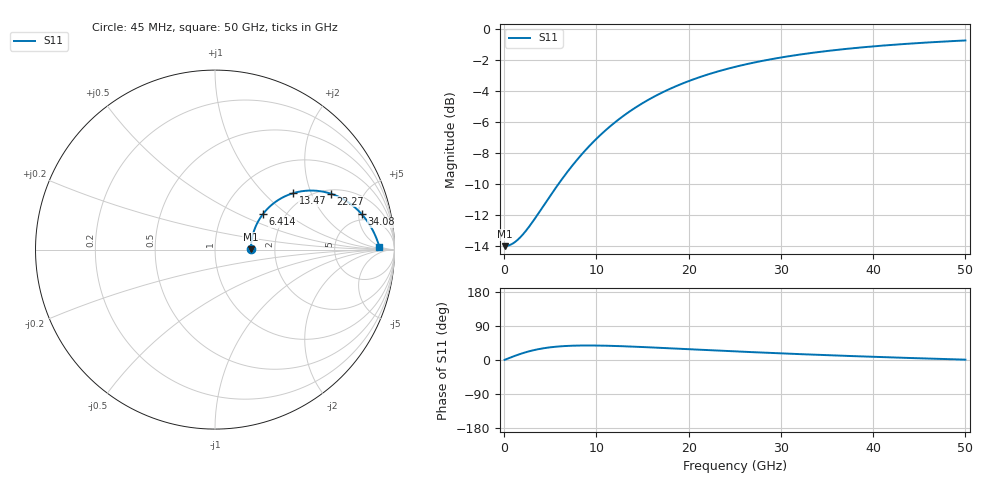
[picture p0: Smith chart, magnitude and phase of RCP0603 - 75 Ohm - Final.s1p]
!Vishay Electro-Films Inc.
!RCP Family
!Case Size 0603
!Assembly Style Surface Mount
!11/2/2015
!efi@vishay.com
# GHz S MA R 50
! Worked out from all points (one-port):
!   801 points, 45 MHz to 50 GHz, reference 50 ohm
!   lowest |S11| = -14.0 dB at 45 MHz (marker M1), VSWR 1.50, Z = 75 + j0.239 ohm
!   |S11| at or under -10 dB: start of sweep to 5.867 GHz
!   S11 on the Smith chart (normalised r, x): 45 MHz: 1.50, +0.00; 6.414 GHz: 1.54, +0.69; 13.47 GHz: 1.71, +1.51; 22.27 GHz: 2.18, +2.78; 34.08 GHz: 4.05, +5.45; 50 GHz: 22, +4
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0.045  0.2 0.4
0.54455  0.2014 5.3
1.0441  0.205 9.9
1.54365  0.2107 14.3
2.105644  0.2195 18.8
2.917413  0.2357 24.3
4.103844  0.2652 30.3
6.289375  0.3291 36.4
6.414263  0.333 36.6
7.850469  0.3774 38.0
9.349119  0.4232 38.3
10.91021  0.469 37.8
12.53375  0.514 36.6
13.47041  0.5385 35.8
14.71928  0.5693 34.5
16.0306  0.5996 33.1
18.77812  0.656 30.0
20.46411  0.6862 28.0
22.27498  0.7153 25.9
25.0225  0.7534 22.8
28.08224  0.7886 19.5
31.26687  0.8187 16.3
34.07684  0.8408 13.6
37.51125  0.8631 10.5
40.57099  0.8796 8.0
43.75563  0.894 5.5
46.87781  0.9059 3.1
50  0.916 0.9
